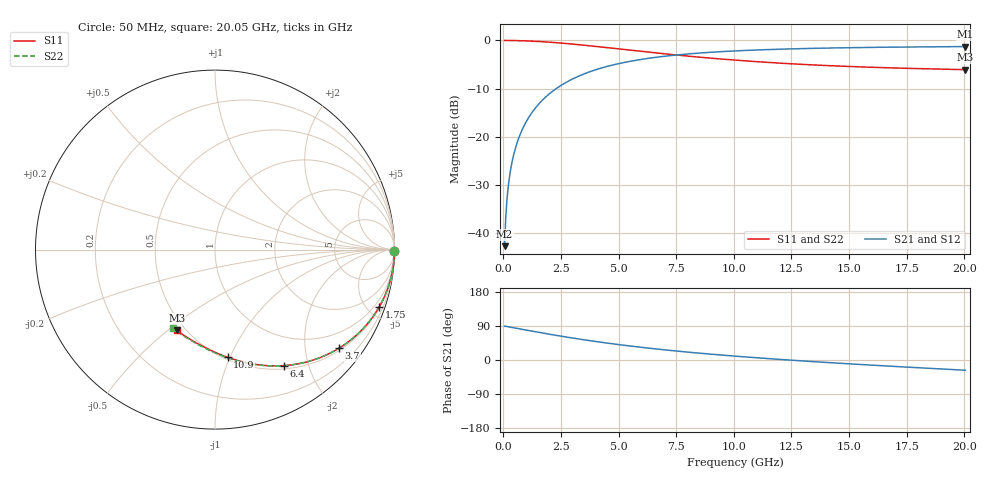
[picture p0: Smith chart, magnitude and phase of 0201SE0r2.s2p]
! AVX Thin Film Operation		Date: August 2001
! Description: Accu-P® Series, Thin Film, SMD, RF Capacitor
! Part Number: 02013J0R2ABW
! 50 MHz  -  20.05 GHz
! Serial Measurements
# mhz S db R 50
!	S11		S21		S12		S22
!	dB	Phase	dB	Phase	dB	Phase	dB	Phase
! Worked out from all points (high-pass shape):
!   401 points, 50 MHz to 20.05 GHz, reference 50 ohm
!   highest |S21| = -1.27 dB at 20.05 GHz (marker M1); lowest = -42.7 dB at 50 MHz (marker M2)
!   |S21| within 3 dB of the highest: 5.562 GHz to end of sweep
!   lowest |S11| = -6.1 dB at 20.05 GHz (marker M3), VSWR 2.98, Z = 22.5 - j26.9 ohm
!   |S11| at or under -10 dB: nowhere
!   |S22| runs from -6.1 to 0.0 dB; largest |S21 - S12| = 8.6e-05
!   S11 on the Smith chart (normalised r, x): 50 MHz: open; 1.75 GHz: 0.56, -5.81; 3.7 GHz: 0.56, -2.77; 6.4 GHz: 0.55, -1.62; 10.9 GHz: 0.52, -0.98; 20.05 GHz: 0.45, -0.54
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50  -0.00 -0.6  -42.66 89.5  -42.66 89.5  -0.00 -0.6
100  -0.00 -1.1  -36.64 88.9  -36.64 88.9  -0.00 -1.1
200  -0.00 -2.3  -30.62 87.8  -30.62 87.8  -0.00 -2.3
250  -0.01 -2.8  -28.68 87.2  -28.68 87.2  -0.01 -2.8
400  -0.01 -4.5  -24.61 85.5  -24.61 85.5  -0.01 -4.5
550  -0.03 -6.2  -21.86 83.8  -21.86 83.8  -0.03 -6.2
750  -0.05 -8.4  -19.19 81.6  -19.19 81.6  -0.05 -8.4
1050  -0.10 -11.8  -16.33 78.2  -16.33 78.2  -0.10 -11.7
1350  -0.17 -15.0  -14.22 74.9  -14.22 74.9  -0.17 -15.0
1750  -0.28 -19.4  -12.10 70.6  -12.10 70.6  -0.28 -19.3
2500  -0.54 -27.1  -9.32 62.9  -9.32 62.9  -0.54 -27.1
3400  -0.94 -35.8  -7.13 54.2  -7.13 54.2  -0.94 -35.7
3700  -1.08 -38.5  -6.57 51.5  -6.57 51.5  -1.08 -38.5
4950  -1.72 -48.9  -4.86 41.0  -4.86 41.0  -1.73 -48.9
6400  -2.48 -59.3  -3.63 30.6  -3.63 30.6  -2.48 -59.4
6750  -2.65 -61.5  -3.41 28.3  -3.41 28.3  -2.65 -61.7
8350  -3.40 -70.9  -2.67 18.8  -2.67 18.8  -3.40 -71.2
10050  -4.08 -79.4  -2.17 10.2  -2.17 10.2  -4.08 -79.9
10900  -4.37 -83.3  -1.99 6.3  -1.99 6.3  -4.38 -83.9
13400  -5.07 -93.4  -1.64 -4.1  -1.64 -4.1  -5.08 -94.5
16750  -5.68 -105.0  -1.39 -16.2  -1.39 -16.2  -5.70 -107.0
20050  -6.05 -115.3  -1.27 -27.1  -1.27 -27.1  -6.08 -118.2
